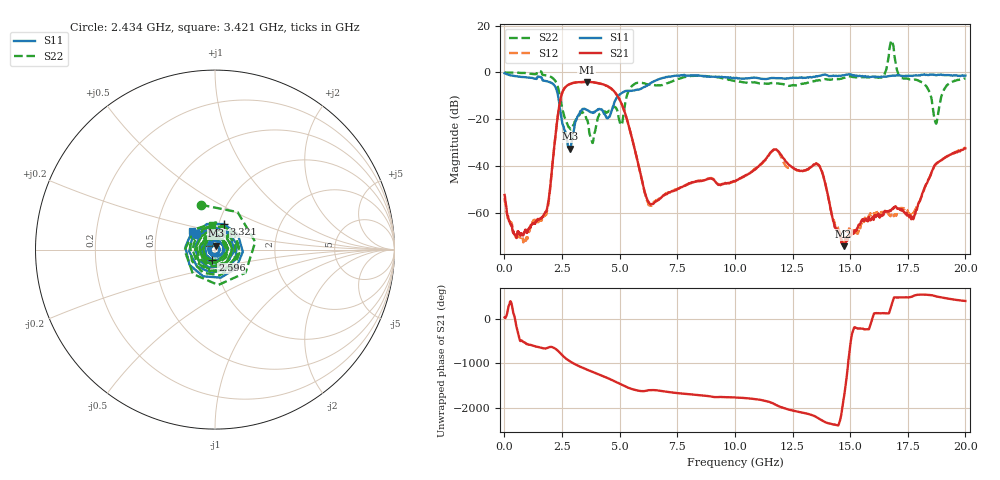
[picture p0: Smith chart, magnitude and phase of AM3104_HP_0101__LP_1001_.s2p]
!Created with skrf (http://scikit-rf.org).
# Hz S RI R 50.0
!freq ReS11 ImS11 ReS21 ImS21 ReS12 ImS12 ReS22 ImS22
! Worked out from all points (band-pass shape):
!   1601 points, 10 MHz to 20 GHz, reference 50 ohm
!   highest |S21| = -4.04 dB at 3.571 GHz (marker M1); lowest = -74.3 dB at 14.72 GHz (marker M2)
!   |S21| within 3 dB of the highest: 2.588 GHz to 4.656 GHz (2.067 GHz wide, 57.1 % of centre)
!   lowest |S11| = -32.6 dB at 2.859 GHz (marker M3), VSWR 1.05, Z = 50.6 + j2.26 ohm
!   |S11| at or under -10 dB: 2.328 GHz to 4.941 GHz (2.613 GHz wide, 71.9 % of centre)
!   |S22| runs from -30.2 to 13.7 dB; largest |S21 - S12| = 0.048
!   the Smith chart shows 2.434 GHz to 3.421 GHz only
!   S11 on the Smith chart (normalised r, x): 2.434 GHz: 0.80, +0.14; 2.596 GHz: 0.96, -0.11; 3.321 GHz: 1.06, +0.31; 3.421 GHz: 0.76, +0.17
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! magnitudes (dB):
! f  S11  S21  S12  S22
! 10 MHz  -0.4  -52.4  -53.7  -0.1
! 459.8 MHz  -1.6  -69.4  -69.8  -0.1
! 1.772 GHz  -3.6  -59.7  -61.2  -1.2
! 2.434 GHz  -17.3  -11.4  -11.5  -11.6
! 2.596 GHz  -24.5  -6.9  -6.9  -18.7
! 2.859 GHz  -32.6  -4.9  -4.9  -24.2
! 3.321 GHz  -16.4  -4.1  -4.2  -17.3
! 3.346 GHz  -16.2  -4.1  -4.2  -16.9
! 3.421 GHz  -15.7  -4.1  -4.1  -17.4
! 3.571 GHz  -16.0  -4.0  -4.1  -20.1
! 3.808 GHz  -17.2  -4.2  -4.2  -29.8
! 4.908 GHz  -10.4  -10.1  -10.1  -16.7
! 6.194 GHz  -5.6  -54.3  -54.9  -5.1
! 6.682 GHz  -3.0  -54.5  -54.3  -5.6
! 10.01 GHz  -2.5  -46.6  -46.5  -3.7
! 11.72 GHz  -2.4  -33.0  -33.1  -4.5
! 13.34 GHz  -2.1  -40.2  -40.1  -4.0
! 14.72 GHz  -1.2  -74.3  -72.5  -2.4
! 16.68 GHz  -1.6  -59.5  -60.8  7.3
! 17.74 GHz  -1.4  -62.8  -60.2  -3.1
! 18.71 GHz  -1.2  -39.1  -39.4  -21.7
! 20 GHz  -1.3  -32.5  -32.2  -2.6
